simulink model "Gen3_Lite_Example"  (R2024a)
settings: Solver=ode1  StartTime=0.0  StopTime=10.0  FixedStep=0.0001  RelTol=1e-3
libraries: Gen3_Lite_Library x5

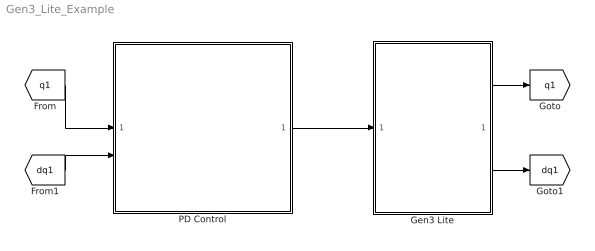
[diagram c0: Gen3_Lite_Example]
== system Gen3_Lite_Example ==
  Gen3 Lite : Subsystem
  PD Control : Subsystem
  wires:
  Gen3 Lite/1(q) -> [q1]
  Gen3 Lite/2(dq) -> [dq1]
  [q1] -> PD Control/1(q)
  [dq1] -> PD Control/2(dq)
  PD Control/1(Tau) -> Gen3 Lite/1(Tau)

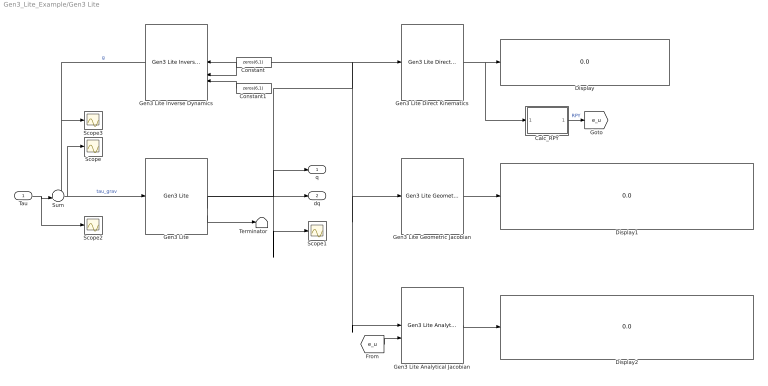
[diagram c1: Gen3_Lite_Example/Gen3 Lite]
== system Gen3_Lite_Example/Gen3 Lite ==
  Tau : Inport
  Calc_RPY : MATLAB Function  TreatAsAtomicUnit=on
  Constant : Constant  Value=zeros(6,1)
  Constant1 : Constant  Value=zeros(6,1)
  Display : Display
  Display1 : Display
  Display2 : Display
  Gen3 Lite : Gen3_Lite_Library/Gen3 Lite  q0=zeros(6,1)  dq0=zeros(6,1)
  Gen3 Lite Analytical Jacobian : Gen3_Lite_Library/Gen3 Lite Analytical Jacobian
  Gen3 Lite Direct Kinematics : Gen3_Lite_Library/Gen3 Lite Direct Kinematics
  Gen3 Lite Geometric Jacobian : Gen3_Lite_Library/Gen3 Lite Geometric Jacobian
  Gen3 Lite Inverse Dynamics : Gen3_Lite_Library/Gen3 Lite Inverse Dynamics
  Scope{,1..3} (4 alike) : Scope
  Sum : Sum  Inputs=++|
  Terminator : Terminator
  q : Outport
  dq : Outport  Port=2
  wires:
  Gen3 Lite Analytical Jacobian/1 -> Display2/1
  Gen3 Lite Direct Kinematics/1 -> Calc_RPY/1(T), Display/1
  Gen3 Lite/1 -> Scope1/1, q/1, Gen3 Lite Inverse Dynamics/1, Gen3 Lite Direct Kinematics/1, Gen3 Lite Geometric Jacobian/1, Gen3 Lite Analytical Jacobian/1
  Gen3 Lite/3 -> Terminator/1
  Gen3 Lite/2 -> dq/1
  Constant/1 -> Gen3 Lite Inverse Dynamics/2
  Gen3 Lite Inverse Dynamics/1 -> Scope3/1, Sum/1  "g"
  Sum/1 -> Gen3 Lite/1, Scope/1  "tau_grav"
  Gen3 Lite Geometric Jacobian/1 -> Display1/1
  Tau/1 -> Scope2/1, Sum/2
  Constant1/1 -> Gen3 Lite Inverse Dynamics/3
  Calc_RPY/1(RPY) -> [e_u]  "RPY"
  [e_u] -> Gen3 Lite Analytical Jacobian/2

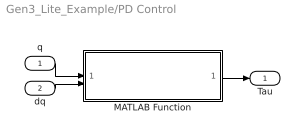
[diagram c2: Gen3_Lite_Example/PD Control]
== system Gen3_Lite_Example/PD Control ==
  q : Inport
  dq : Inport  Port=2
  MATLAB Function : MATLAB Function  TreatAsAtomicUnit=on
  Tau : Outport
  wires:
  MATLAB Function/1(tau) -> Tau/1
  q/1 -> MATLAB Function/1(q)
  dq/1 -> MATLAB Function/2(dq)

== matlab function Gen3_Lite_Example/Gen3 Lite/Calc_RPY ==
function RPY = calc_RPY(T)
R=T(1:3,1:3);
p=T(1:3,4);

r31=R(3,1);
r32=R(3,2);
r33=R(3,3);
r21=R(2,1);
r11=R(1,1);

theta=atan2(-r31,sqrt(r32^2+r33^2));
psi=atan2(r32/cos(theta),r33/cos(theta));
phi=atan2(r21/cos(theta),r11/cos(theta));
RPY=[psi;theta;phi];

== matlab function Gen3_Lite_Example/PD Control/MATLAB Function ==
function tau = PD_Control(q,dq)

kp=diag([2,2,2,2,2,2]);
kd=diag([1,1,1,1,1,1]);
qd=[0;pi/2;0;-pi/2;pi/3;pi/4];

tau = -kp*(q-qd)-kd*dq;
